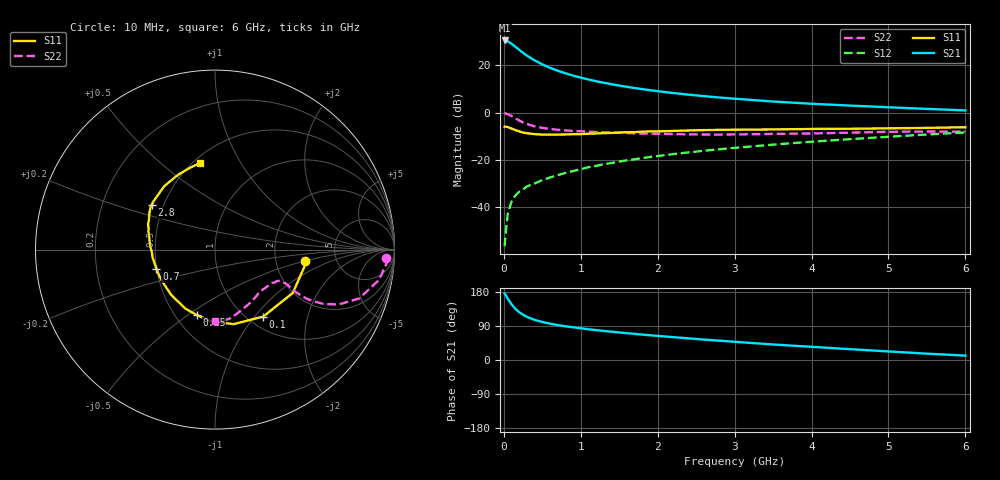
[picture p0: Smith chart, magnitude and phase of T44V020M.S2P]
! Infineon Technologies  Discrete & RF Semiconductors
! BFR182T
! Si NPN RF Bipolar Junction Transistor in SC75
! VCE = 4 V  IC = 20 mA
! Common Emitter S-Parameters:  October  1999
# GHz  S  MA  R  50
!  f  S11  S21  S12  S22
! GHz  MAG  ANG  MAG  ANG  MAG  ANG  MAG  ANG
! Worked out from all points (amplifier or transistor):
!   36 points, 10 MHz to 6 GHz, reference 50 ohm
!   highest |S21| = 30.5 dB at 10 MHz (marker M1)
!   |S21| within 3 dB of that: start of sweep to 163 MHz
!   unconditionally stable (mu >= 1): 670.1 MHz to 3.659 GHz
!   at 250 MHz: K = 0.66, MSG = 28.9 dB, |S12| = -32.5 dB
!   at 1.4 GHz: K = 1.10, MAG = 14.7 dB, |S12| = -21.3 dB
!   at 6 GHz: K = 0.84, MSG = 4.7 dB, |S12| = -8.4 dB
!   S11 on the Smith chart (normalised r, x): 10 MHz: 2.94, -0.49; 100 MHz: 1.17, -1.11; 250 MHz: 0.64, -0.54; 700 MHz: 0.50, -0.12; 2.8 GHz: 0.43, +0.26; 6 GHz: 0.54, +0.69
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0.01  0.5042 -7.0  33.62 175.1  0.0015 89.9  0.955 -2.8
0.02  0.5082 -10.3  33.34 172.7  0.0024 101.5  0.9618 -4.2
0.05  0.4963 -29.1  32.27 162.0  0.0071 85.9  0.9288 -10.5
0.1  0.4598 -54.2  28.64 147.0  0.0131 74.7  0.8488 -18.7
0.15  0.428 -75.9  24.75 134.9  0.0177 66.8  0.7558 -23.8
0.2  0.4019 -92.5  21.3 126.0  0.0213 66.2  0.6814 -26.5
0.25  0.3784 -105.6  18.41 119.3  0.0237 62.2  0.6203 -27.7
0.3  0.3678 -116.8  16.09 113.9  0.0275 63.5  0.5766 -28.2
0.4  0.351 -134.0  12.75 105.9  0.0318 63.5  0.5122 -27.8
0.5  0.3433 -145.6  10.5 100.4  0.0374 65.8  0.4764 -26.7
0.6  0.3427 -154.4  8.869 95.9  0.0425 67.2  0.4521 -26.1
0.7  0.3441 -161.8  7.706 92.2  0.0477 67.7  0.4335 -25.6
0.9  0.3505 -172.6  6.072 86.3  0.0583 70.4  0.4093 -25.5
1.1  0.3583 178.6  5.023 81.1  0.0703 70.5  0.3961 -26.2
1.3  0.3685 172.0  4.289 76.7  0.0814 71.2  0.3838 -27.6
1.6  0.386 164.2  3.51 70.7  0.0981 71.1  0.3703 -30.0
2.2  0.4102 153.5  2.603 60.3  0.1325 70.4  0.3525 -37.2
2.8  0.4319 144.8  2.092 51.0  0.1679 68.4  0.3433 -45.4
3.5  0.4412 135.2  1.719 40.9  0.2105 65.5  0.3549 -55.6
4.5  0.4561 122.9  1.41 28.6  0.2749 60.3  0.3773 -71.1
5.5  0.4758 107.3  1.201 16.7  0.3449 54.2  0.3985 -84.2
6  0.4914 99.5  1.115 11.6  0.3808 50.5  0.3981 -89.6
